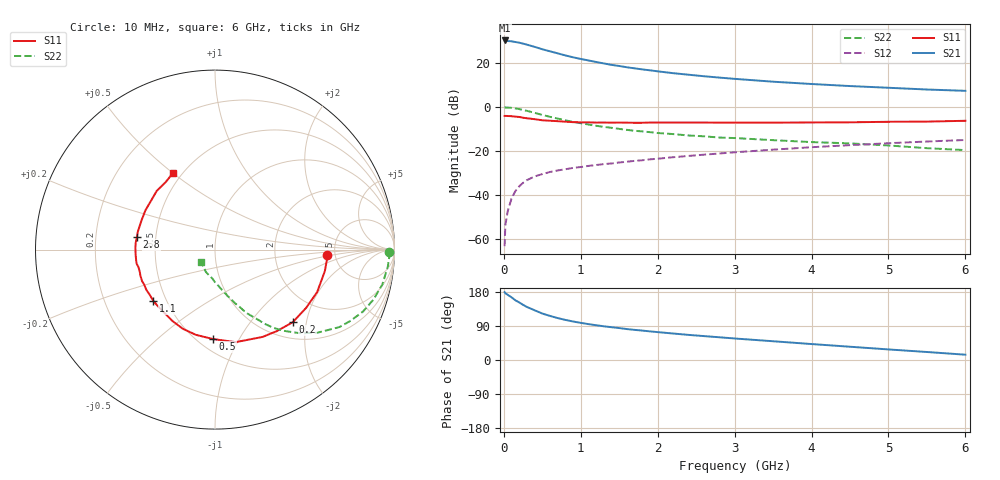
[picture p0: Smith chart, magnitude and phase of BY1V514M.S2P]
! SIEMENS Small Signal Semiconductors
! BFY420
! Si NPN RF SIEGET Grounded Emitter Transistor in MICRO-X
! VCE = 1.5 V  IC = 14 mA
! Common Emitter S-Parameters:  October  1996
# GHz  S  MA  R  50
!  f  S11  S21  S12  S22
! GHz  MAG  ANG  MAG  ANG  MAG  ANG  MAG  ANG
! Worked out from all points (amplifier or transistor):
!   36 points, 10 MHz to 6 GHz, reference 50 ohm
!   highest |S21| = 30.1 dB at 10 MHz (marker M1)
!   |S21| within 3 dB of that: start of sweep to 410 MHz
!   unconditionally stable (mu >= 1): 2.176 GHz to end of sweep
!   at 250 MHz: K = 0.24, MSG = 31.5 dB, |S12| = -34.4 dB
!   at 1.4 GHz: K = 0.85, MSG = 22.3 dB, |S12| = -25.6 dB
!   at 6 GHz: K = 1.09, MAG = 9.3 dB, |S12| = -15.0 dB
!   S11 on the Smith chart (normalised r, x): 10 MHz: 4.30, -0.42; 200 MHz: 1.34, -1.67; 500 MHz: 0.59, -0.78; 1.1 GHz: 0.42, -0.31; 2.8 GHz: 0.39, +0.07; 6 GHz: 0.45, +0.50
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0.01  0.6259 -2.7  32.09 179.0  0.0007 94.6  0.9671 -0.8
0.02  0.6262 -5.0  32.03 176.2  0.0021 85.2  0.9729 -2.0
0.05  0.6237 -11.1  31.14 172.0  0.0043 83.2  0.9674 -5.7
0.1  0.6164 -22.6  30.68 165.5  0.0084 79.6  0.9524 -11.8
0.15  0.6027 -32.5  29.57 157.6  0.0124 74.3  0.9257 -17.5
0.2  0.5928 -43.1  28.57 151.9  0.0159 71.0  0.894 -22.7
0.25  0.5698 -52.9  27.21 145.5  0.0191 68.0  0.8531 -27.7
0.3  0.5541 -61.4  25.79 140.0  0.022 65.9  0.8167 -31.9
0.4  0.5283 -77.4  23.01 131.2  0.0266 60.2  0.7346 -39.1
0.5  0.4985 -91.3  20.29 122.6  0.0301 57.3  0.6601 -44.8
0.6  0.4867 -102.7  18.21 116.3  0.0336 55.4  0.597 -49.4
0.7  0.4759 -112.2  16.39 110.6  0.0364 54.1  0.5448 -53.2
0.8  0.4629 -120.9  14.7 105.8  0.0387 51.3  0.4975 -56.2
0.9  0.4522 -127.7  13.33 101.6  0.0416 51.4  0.4591 -58.4
1.1  0.4474 -140.0  11.3 94.7  0.0461 51.2  0.3998 -63.1
1.6  0.4404 -160.6  7.923 81.6  0.0574 50.6  0.3021 -70.9
2.2  0.4431 -177.1  5.823 69.9  0.0725 50.1  0.2427 -78.1
2.8  0.4407 170.8  4.627 60.0  0.0881 47.7  0.2027 -84.5
3.5  0.4406 158.4  3.731 49.5  0.1077 43.8  0.1767 -91.3
4.5  0.4483 142.8  2.972 35.0  0.1363 36.3  0.1493 -101.8
5.5  0.4654 126.3  2.482 21.1  0.1646 27.4  0.1163 -122.3
6  0.4856 119.1  2.318 14.0  0.1783 22.7  0.1051 -137.5
